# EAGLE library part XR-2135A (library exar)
Bell/CCITT type data BUFFER
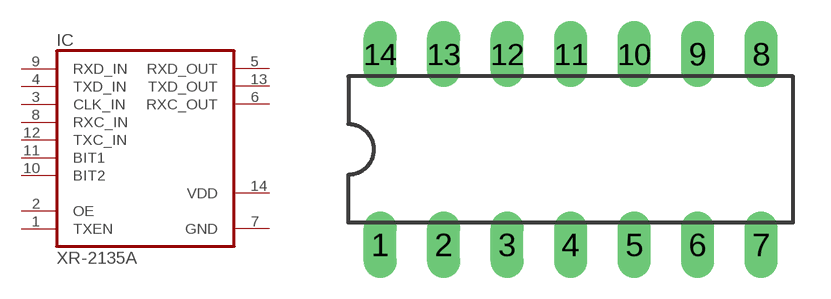
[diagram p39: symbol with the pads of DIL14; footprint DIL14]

Designator prefix IC

## XR-2135A (OC_FARNELL: unknown; OC_NEWARK: unknown)  [DIL14]
1  TXEN  in
2  OE  in
3  CLK_IN  in
4  TXD_IN  in
5  RXD_OUT  out
6  RXC_OUT  out
7  GND  pwr
8  RXC_IN  in
9  RXD_IN  in
10  BIT2  in
11  BIT1  in
12  TXC_IN  in
13  TXD_OUT  out
14  VDD  pwr

## Footprint DIL14 (pad centres in mm)
Dual In Line Package
drill 0.813 long: 1 -7.62,-3.81; 2 -5.08,-3.81; 3 -2.54,-3.81; 4 0,-3.81; 5 2.54,-3.81; 6 5.08,-3.81; 7 7.62,-3.81; 8 7.62,3.81; 9 5.08,3.81; 10 2.54,3.81; 11 0,3.81; 12 -2.54,3.81; 13 -5.08,3.81; 14 -7.62,3.81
